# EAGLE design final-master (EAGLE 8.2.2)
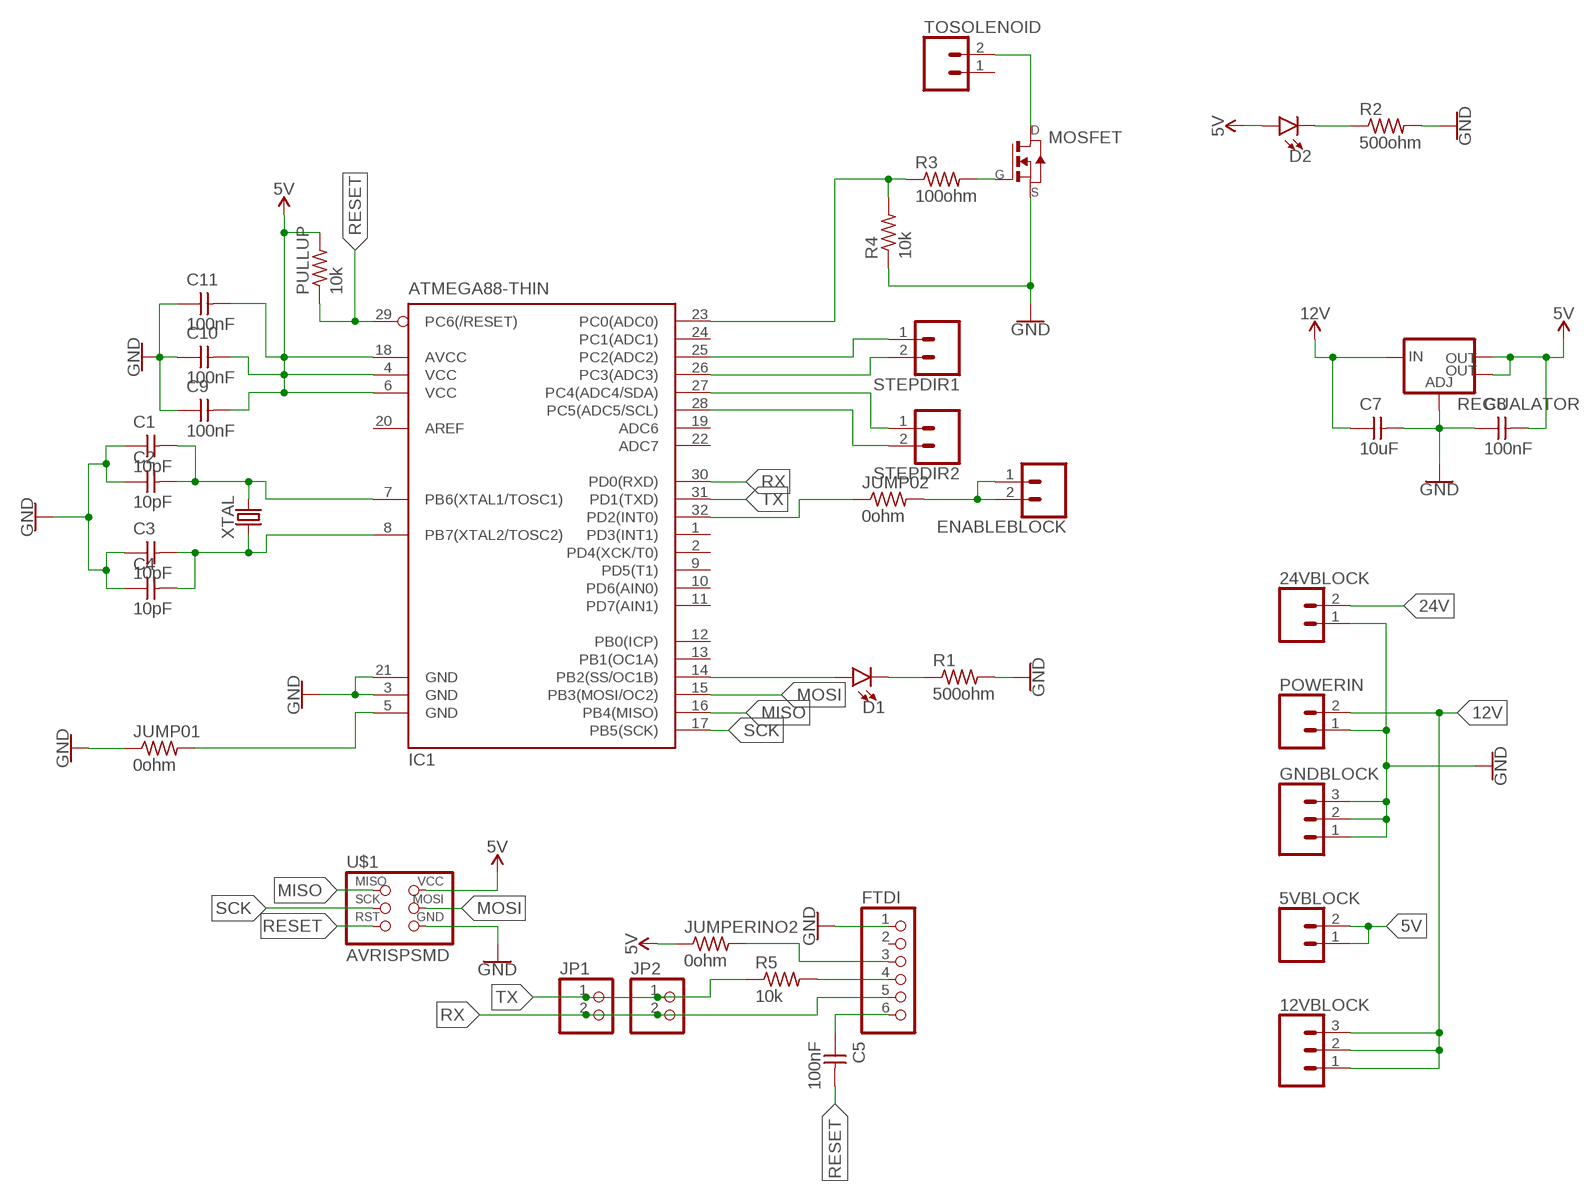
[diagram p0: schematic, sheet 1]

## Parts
5VBLOCK  CONN_023.5MM_LOCK  [SCREWTERMINAL-3.5MM-2_LOCK]
12VBLOCK  CONN_03SCREW_LOCK  [SCREWTERMINAL-3.5MM-3_LOCK.007S]
24VBLOCK  CONN_023.5MM_LOCK  [SCREWTERMINAL-3.5MM-2_LOCK]
C1  10pF  CAP-UNPOLARIZEDFAB  [C1206FAB]
C2  10pF  CAP-UNPOLARIZEDFAB  [C1206FAB]
C3  10pF  CAP-UNPOLARIZEDFAB  [C1206FAB]
C4  10pF  CAP-UNPOLARIZEDFAB  [C1206FAB]
C5  100nF  CAP-UNPOLARIZEDFAB  [C1206FAB]
C7  10uF  CAP-UNPOLARIZEDFAB  [C1206FAB]
C8  100nF  CAP-UNPOLARIZEDFAB  [C1206FAB]
C9  100nF  CAP-UNPOLARIZEDFAB  [C1206FAB]
C10  100nF  CAP-UNPOLARIZEDFAB  [C1206FAB]
C11  100nF  CAP-UNPOLARIZEDFAB  [C1206FAB]
D1  LED1206  [LED-1206]
D2  LED1206  [LED-1206]
ENABLEBLOCK  CONN_023.5MM_LOCK  [SCREWTERMINAL-3.5MM-2_LOCK]
FTDI  PINHD-1X6  [1X06]
GNDBLOCK  CONN_03SCREW_LOCK  [SCREWTERMINAL-3.5MM-3_LOCK.007S]
IC1  ATMEGA88-THIN  [TQFP32-08THIN]
JP1  PINHD-1X2  [1X02]
JP2  PINHD-1X2  [1X02]
JUMP01  0ohm  RES-US1206FAB  [R1206FAB]
JUMP02  0ohm  RES-US1206FAB  [R1206FAB]
JUMPERINO2  0ohm  RES-US1206FAB  [R1206FAB]
MOSFET  STN3NF06L  [SOT223]
POWERIN  CONN_023.5MM  [SCREWTERMINAL-3.5MM-2]
PULLUP  10k  RES-US1206FAB  [R1206FAB]
R1  500ohm  RES-US1206FAB  [R1206FAB]
R2  500ohm  RES-US1206FAB  [R1206FAB]
R3  100ohm  RES-US1206FAB  [R1206FAB]
R4  10k  RES-US1206FAB  [R1206FAB]
R5  10k  RES-US1206FAB  [R1206FAB]
REGUALATOR  V_REG_LM1117SOT223  [SOT223]
STEPDIR1  CONN_023.5MM_LOCK  [SCREWTERMINAL-3.5MM-2_LOCK]
STEPDIR2  CONN_023.5MM_LOCK  [SCREWTERMINAL-3.5MM-2_LOCK]
TOSOLENOID  CONN_023.5MM  [SCREWTERMINAL-3.5MM-2]
U$1  AVRISPSMD  [2X03SMD]
XTAL  CRYSTALSMD-HC49UP  [HC49UP]

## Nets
5V: 5VBLOCK.1 5VBLOCK.2 C8.2 C9.2 C10.2 C11.2 D2.A IC1.4(VCC) IC1.6(VCC) IC1.18(AVCC) JUMPERINO2.1 PULLUP.2 REGUALATOR.2(OUT) REGUALATOR.4(OUT) U$1.2(VCC)
12V: 12VBLOCK.1 12VBLOCK.2 12VBLOCK.3 C7.1 POWERIN.2 REGUALATOR.3(IN)
24V: 24VBLOCK.2
DIR1: IC1.26(PC3(ADC3)) STEPDIR1.2
DIR2: IC1.27(PC4(ADC4/SDA)) STEPDIR2.1
DRAIN: MOSFET.2(D) MOSFET.4(D) TOSOLENOID.2
ENABLEPIN: IC1.32(PD2(INT0)) JUMP02.1
GATE: MOSFET.1(G) R3.2
GND: 24VBLOCK.1 C1.1 C2.1 C3.1 C4.1 C7.2 C8.1 C9.1 C10.1 C11.1 FTDI.1 GNDBLOCK.1 GNDBLOCK.2 GNDBLOCK.3 IC1.3(GND) IC1.5(GND) IC1.21(GND) JUMP01.1 JUMP01.2 MOSFET.3(S) POWERIN.1 R1.2 R2.2 R4.1 REGUALATOR.1(ADJ) U$1.6(GND)
MISO: IC1.16(PB4(MISO)) U$1.1(MISO)
MOSI: IC1.15(PB3(MOSI/OC2)) U$1.4(MOSI)
N$1: C3.2 C4.2 IC1.8(PB7(XTAL2/TOSC2)) XTAL.1
N$2: C1.2 C2.2 IC1.7(PB6(XTAL1/TOSC1)) XTAL.2
N$3: IC1.23(PC0(ADC0)) R3.1 R4.2
N$4: ENABLEBLOCK.1 ENABLEBLOCK.2 JUMP02.2
N$6: D1.A IC1.14(PB2(SS/OC1B))
N$7: FTDI.3 JUMPERINO2.2
N$8: C5.1 FTDI.6
N$12: FTDI.4 R5.2
N$23: D2.C R2.1
N$26: D1.C R1.1
RESET: C5.2 IC1.29(PC6(/RESET)) PULLUP.1 U$1.5(RST)
RX: FTDI.5 IC1.30(PD0(RXD)) JP1.2 JP2.2
SCK: IC1.17(PB5(SCK)) U$1.3(SCK)
STEP1: IC1.25(PC2(ADC2)) STEPDIR1.1
STEP2: IC1.28(PC5(ADC5/SCL)) STEPDIR2.2
TX: IC1.31(PD1(TXD)) JP1.1 JP2.1 R5.1
Unconnected: FTDI.2 IC1.1(PD3(INT1)) IC1.2(PD4(XCK/T0)) IC1.9(PD5(T1)) IC1.10(PD6(AIN0)) IC1.11(PD7(AIN1)) IC1.12(PB0(ICP)) IC1.13(PB1(OC1A)) IC1.19(ADC6) IC1.20(AREF) IC1.22(ADC7) IC1.24(PC1(ADC1)) TOSOLENOID.1

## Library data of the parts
5VBLOCK 24VBLOCK ENABLEBLOCK POWERIN STEPDIR1 STEPDIR2 TOSOLENOID = SparkFun-Connectors:CONN_02: Multi connection point. Often used as Generic Header-pin footprint for 0.1 inch spaced/style header connections; PROD_ID: CONN-08399
12VBLOCK GNDBLOCK = SparkFun-Connectors:CONN_03: Multi connection point. Often used as Generic Header-pin footprint for 0.1 inch spaced/style header connections On any of the 0.1 inch spaced packages, you can populate with these: Break Away Headers - Straight (PRT-00116) Break Away Male Headers - Right Angle (PRT-00553) Female Headers (PRT-00115)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; PROD_ID: CONN-08288; SF_ID: PRT-08235
C1-C5 C7-C11 = 01fab:CAP-UNPOLARIZED
D1 D2 = SparkFun-LED:LED: LED (Generic)
FTDI = pinhead:PINHD-1X6: PIN HEADER
IC1 = 01fab:ATMEGA88-THIN
JP1 JP2 = pinhead:PINHD-1X2: PIN HEADER
JUMP01 JUMP02 JUMPERINO2 PULLUP R1-R5 = 01fab:RES-US: Resistor (US Symbol)
MOSFET = 01guercio:STN3NF06L
REGUALATOR = 01fab:V_REG_LM1117: Voltage Regulator LM1117 Standard adjustable voltage regulator but in SMD form. Spark Fun Electronics SKU : COM-00595; PROD_ID: VREG-08170
U$1 = 01fab:AVRISP
XTAL = SparkFun-Clocks:CRYSTAL: Crystals (Generic)

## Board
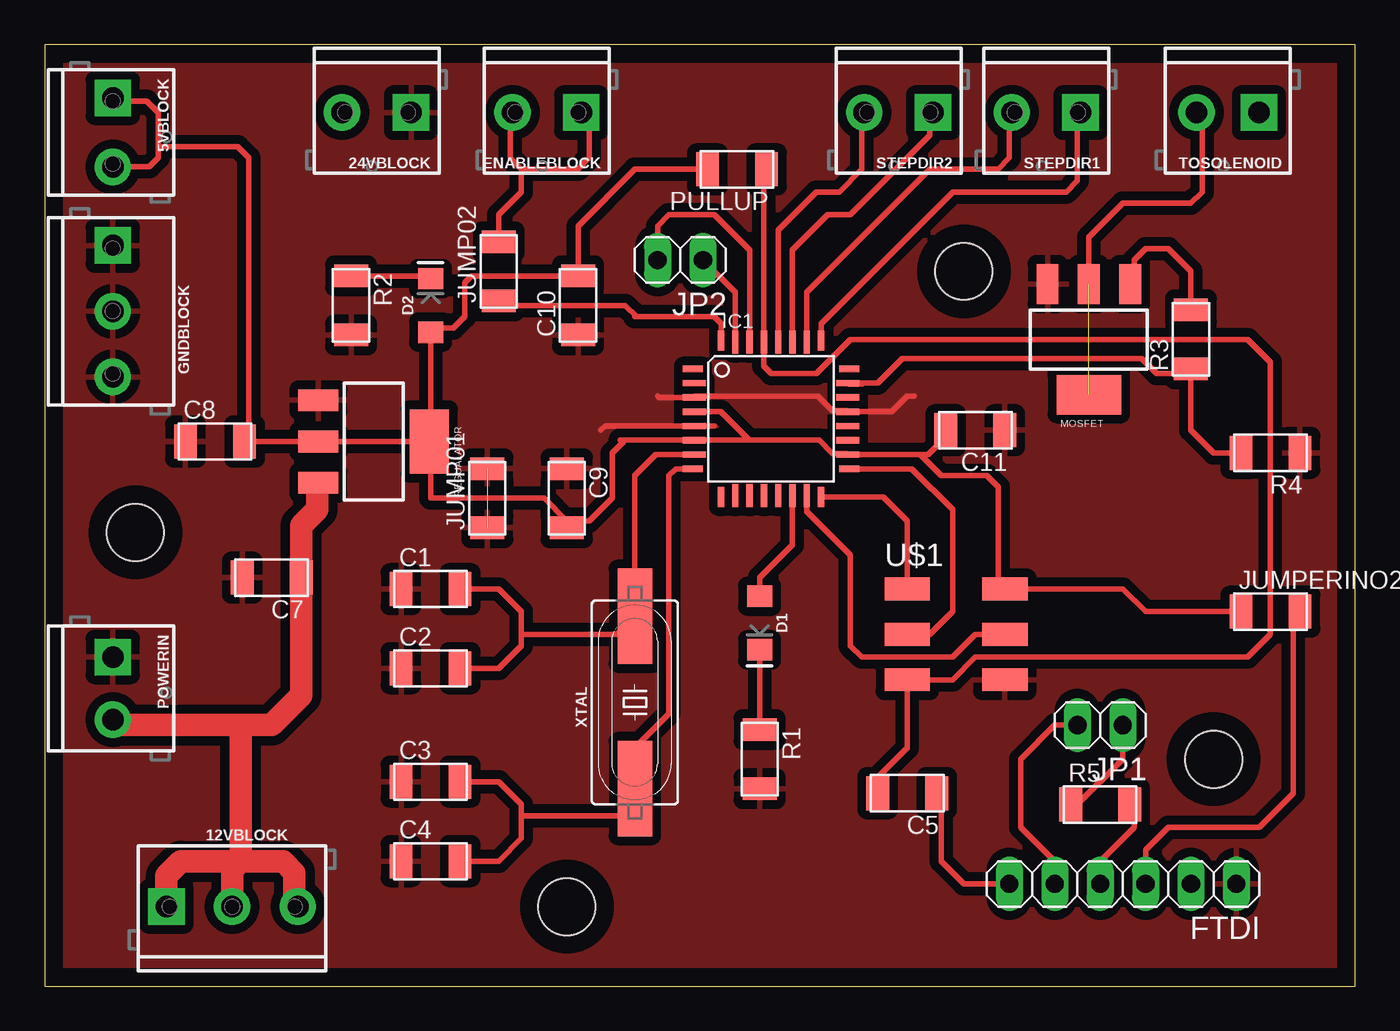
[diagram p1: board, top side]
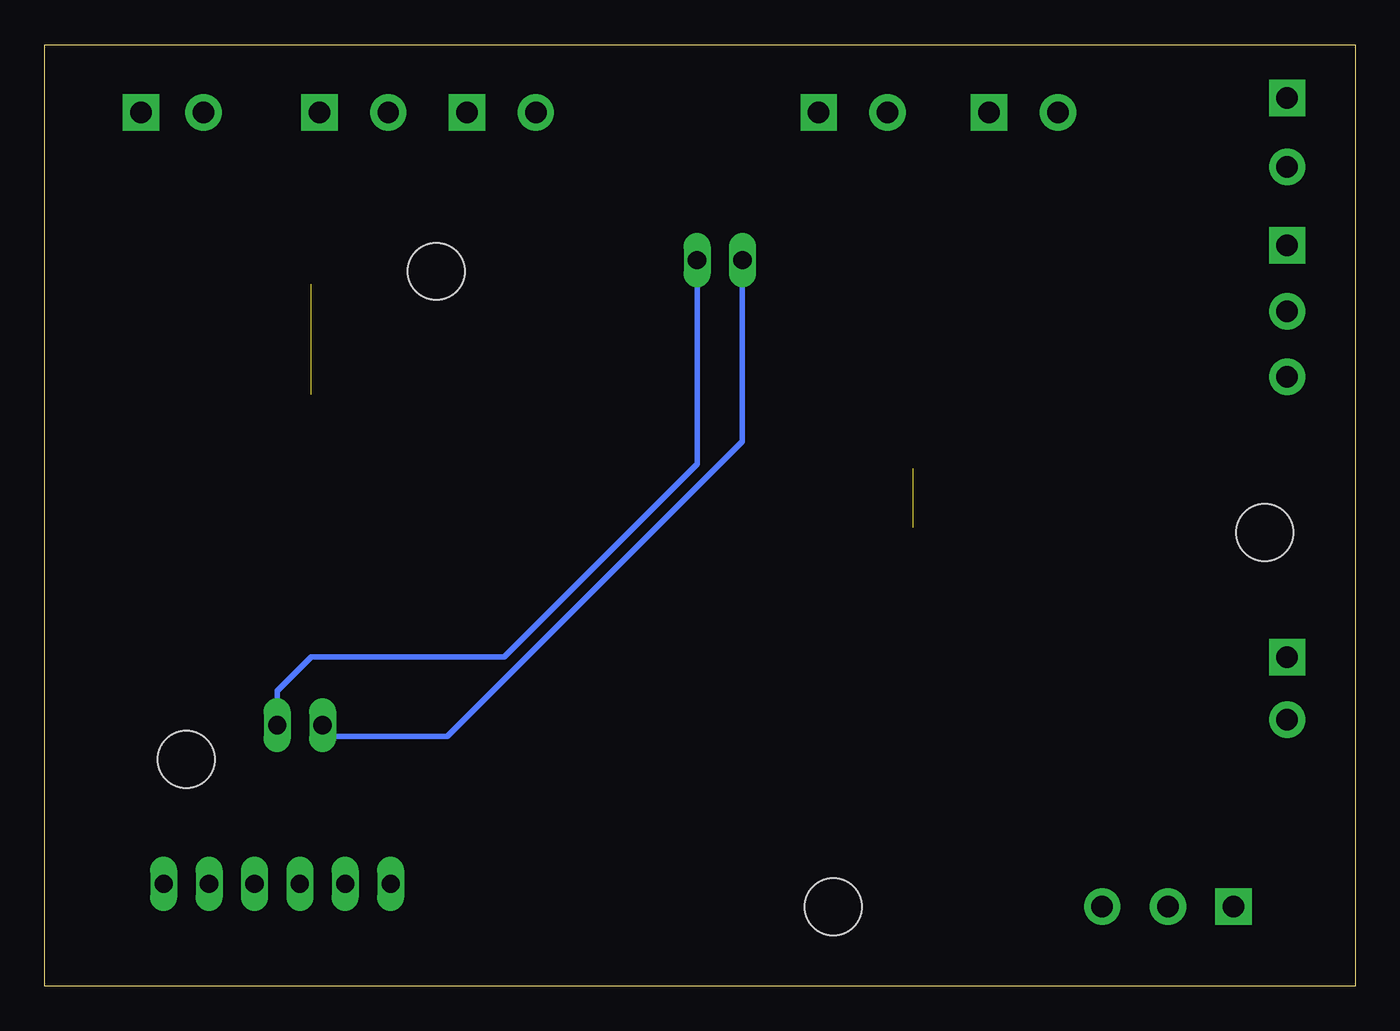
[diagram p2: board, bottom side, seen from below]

Size 73.33 x 52.7 mm. Coordinates in mm from the lower left corner, seen from the top.
Outline: 0,0 73.33,0 73.33,52.7 0,52.7 0,0
Copper layers (1*16): Top 0.035mm / dielectric 1.5mm / Bottom 0.035mm
Design rules "default *": minimum track width 12mil, minimum drill 0.35mm, track to track 16mil, track to pad 16mil, pad to pad 16mil, via to via 16mil, smd to smd 16mil, copper to edge 40mil, drill to drill 6mil, minimum pad ring 10mil, minimum via ring 8mil, stop-mask expansion 4mil, vias tented up to drill 0mil, thermal gap 20mil
Holes 3.2 mm at 51.44,40.01 29.21,4.45 65.41,12.7 5.08,25.4

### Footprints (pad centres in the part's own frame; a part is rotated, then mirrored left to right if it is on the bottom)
SCREWTERMINAL-3.5MM-2_LOCK = drill 1.2 pad 2.032 square: 1 -0.178,0 | drill 1.2 pad 2.032: 2 3.678,0
SCREWTERMINAL-3.5MM-3_LOCK.007S = drill 1.2 pad 2.032 square: 1 -0.178,0 | drill 1.2 pad 2.032: 2 3.5,0; 3 7.178,0
C1206FAB = smd 1.27 x 1.905: 1 -1.651,0; 2 1.651,0
LED-1206 = smd 1.2 x 1.4: A -1.5,0; C 1.5,0
1X06 = drill 1.016 long: 1 -6.35,0; 2 -3.81,0; 3 -1.27,0; 4 1.27,0; 5 3.81,0; 6 6.35,0
TQFP32-08THIN = smd 1.118 x 0.356: 1 -4.369,2.8; 8 -4.369,-2.8; 17 4.369,-2.8; 24 4.369,2.8 | smd 1.27 x 0.356: 2 -4.293,2; 3 -4.293,1.2; 4 -4.293,0.4; 5 -4.293,-0.4; 6 -4.293,-1.2; 7 -4.293,-2; 18 4.293,-2; 19 4.293,-1.2; 20 4.293,-0.4; 21 4.293,0.4; 22 4.293,1.2; 23 4.293,2 | smd 0.356 x 1.118: 9 -2.8,-4.369; 16 2.8,-4.369; 25 2.8,4.369; 32 -2.8,4.369 | smd 0.356 x 1.27: 10 -2,-4.293; 14 1.2,-4.293; 15 2,-4.293; 26 2,4.293; 27 1.2,4.293; 31 -2,4.293 | smd 0.35 x 1.27: 11 -1.2,-4.293; 12 -0.4,-4.293; 13 0.4,-4.293; 28 0.4,4.293; 29 -0.4,4.293; 30 -1.2,4.293
1X02 = drill 1.016 long: 1 -1.27,0; 2 1.27,0
R1206FAB = smd 1.27 x 1.905: 1 -1.651,0; 2 1.651,0
SOT223 = smd 1.219 x 2.235: 1 -2.311,-3.099; 2 0,-3.099; 3 2.311,-3.099 | smd 3.6 x 2.2: 4 0,3.099
SCREWTERMINAL-3.5MM-2 = drill 1.2 pad 2.032 square: 1 0,0 | drill 1.2 pad 2.032: 2 3.5,0
2X03SMD = smd 2.54 x 1.27: 1 -2.54,2.54; 2 2.92,2.54; 3 -2.54,0; 4 2.92,0; 5 -2.54,-2.54; 6 2.92,-2.54
HC49UP = smd 5.334 x 1.93: 1 -4.826,0; 2 4.826,0

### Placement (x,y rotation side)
5VBLOCK  3.81,49.53 270 top
12VBLOCK  6.99,4.45 0 top
24VBLOCK  20.32,48.9 180 top
C1  21.59,22.23 0 top
C2  21.59,17.78 0 top
C3  21.59,11.43 0 top
C4  21.59,6.99 0 top
C5  48.26,10.79 180 top
C7  12.7,22.86 180 top
C8  9.53,30.48 0 top
C9  29.21,27.3 270 top
C10  29.84,38.1 90 top
C11  52.07,31.11 180 top
D1  40.01,20.32 270 top
D2  21.59,38.1 90 top
ENABLEBLOCK  29.84,48.9 180 top
FTDI  60.33,5.71 180 top
GNDBLOCK  3.81,41.27 270 top
IC1  40.64,31.75 0 top
JP1  59.05,14.61 180 top
JP2  35.56,40.64 180 top
JUMP01  24.77,27.3 90 top
JUMP02  25.4,40.01 90 top
JUMPERINO2  68.58,20.95 0 top
MOSFET  58.42,36.2 180 top
POWERIN  3.81,18.41 270 top
PULLUP  38.73,45.72 180 top
R1  40.01,12.7 270 top
R2  17.14,38.1 270 top
R3  64.14,36.2 90 top
R4  68.58,29.84 180 top
R5  59.05,10.16 0 top
REGUALATOR  18.41,30.48 270 top
STEPDIR1  57.78,48.9 180 top
STEPDIR2  49.53,48.9 180 top
TOSOLENOID  67.94,48.9 180 top
U$1  50.8,19.68 0 top
XTAL  33.02,15.88 90 top

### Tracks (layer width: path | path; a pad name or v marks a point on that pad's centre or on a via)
5V
  Top 0.305: 32.2,30.55 32.38,30.55 | 32.38,30.55 IC1.6 39.41,30.55 | REGUALATOR.4 21.59,30.4 21.59,27.3 27.94,27.3 29.21,26.04 C9.2 29.59,26.04 30.48,26.04 31.75,27.3 31.75,29.84 32.38,30.48 32.38,30.55 | 39.41,30.55 43.33,30.55 44.07,29.81 44.87,29.81 IC1.18 48.99,29.75 | 48.99,29.75 49.44,29.75 50.16,30.48 50.16,30.86 C11.2 | REGUALATOR.4 21.59,30.56 D2.A 21.82,36.83 22.86,36.83 23.5,37.47 23.5,39.37 23.88,39.75 C10.2 29.84,42.55 33.02,45.72 PULLUP.2 | 48.99,29.75 50.16,28.57 52.7,28.57 53.34,27.94 53.34,22.61 U$1.2 60.33,22.23 61.59,20.95 JUMPERINO2.1 | 5VBLOCK.2 5.85,45.85 6.35,46.35 6.35,46.99 | 6.35,46.99 6.35,48.9 5.71,49.53 3.99,49.53 5VBLOCK.1 | 6.35,46.99 10.79,46.99 11.43,46.35 11.43,30.73 C8.2 REGUALATOR.2 REGUALATOR.4 | IC1.4 37.81,32.15 39.41,30.55
12V
  Top 1.27: 10.85,14.61 12.7,14.61 14.35,16.26 C7.1 14.35,25.78 15.24,26.67 15.24,28.09 REGUALATOR.3 | 10.85,14.61 4.12,14.61 POWERIN.2 | 12VBLOCK.1 6.81,6.17 7.62,6.99 10.98,6.99 | 12VBLOCK.3 13.97,4.64 13.97,6.35 13.34,6.99 10.98,6.99 | 12VBLOCK.2 10.48,6.49 10.98,6.99 | 10.98,6.99 10.98,14.47 10.85,14.61
DIR1
  Top 0.305: IC1.26 42.64,38.83 49.53,45.72 53.34,45.72 53.98,46.35 53.98,48.76 STEPDIR1.2
DIR2
  Top 0.305: IC1.27 41.84,41.2 43.81,43.18 45.09,43.18 49.53,47.62 49.53,48.72 STEPDIR2.1
DRAIN  (1 unrouted)
  Top 0.305: MOSFET.2 58.42,41.91 60.33,43.81 64.14,43.81 64.77,44.45 64.77,48.57 TOSOLENOID.2
ENABLEPIN
  Top 0.305: IC1.32 37.84,37.09 37.47,37.47 33.12,37.47 | 33.12,37.47 33.02,37.47 | JUMP02.1 25.65,38.1 32.48,38.1 33.12,37.47
GATE
  Top 0.305: R3.2 64.14,40.01 62.87,41.27 61.59,41.27 60.96,40.64 60.96,39.52 MOSFET.1
GND  (1 unrouted)
  Top 0.305: 48.64,33.02 48.26,33.02 47.39,32.15 IC1.21 44.87,32.21 44.07,32.21 43.26,33.02 37.22,33.02 37.21,33.01 36.41,33.01 IC1.3 34.36,32.95 34.29,33.02 | 37.45,31.35 IC1.5 31.35,31.35 31.11,31.11
  pour Top (isolate 0.508): -2.54,-2.54 102.23,-2.54 102.87,-1.91 102.87,82.55 103.5,83.19 -2.54,83.19
MISO
  Top 0.305: IC1.16 46.91,27.38 48.26,26.04 U$1.1
MOSI
  Top 0.305: IC1.15 42.64,26.57 45.09,24.13 45.09,19.05 45.72,18.41 50.8,18.41 52.07,19.68 U$1.4
N$1
  Top 0.305: IC1.8 35.3,28.95 34.92,28.57 34.92,15.24 33.02,13.34 XTAL.1 33.02,9.53 26.67,9.53 | C4.2 25.4,6.99 26.67,8.26 26.67,9.53 | 26.67,9.53 26.67,10.16 25.4,11.43 C3.2
N$2
  Top 0.305: IC1.7 34.2,29.75 33.02,28.57 XTAL.2 32,19.68 26.67,19.68 | C1.2 25.4,22.23 26.67,20.95 26.67,19.68 | 26.67,19.68 26.67,19.05 25.4,17.78 C2.2
N$3
  Top 0.305: 45.75,33.69 45,33.69 IC1.23 46.6,33.75 47.99,35.14 61.38,35.14 62.23,34.29 63.88,34.29 R3.1 64.14,31.11 65.41,29.84 R4.2
N$4
  Top 0.305: 26.84,45.72 26.67,45.72 26.04,46.35 26.04,48.76 ENABLEBLOCK.2 | 26.84,45.72 29.84,45.72 30.48,46.35 30.48,48.44 ENABLEBLOCK.1 | 26.84,45.72 26.67,45.55 26.67,44.45 25.4,43.18 JUMP02.2
N$6
  Top 0.305: IC1.14 41.84,24.7 40.01,22.86 D1.A
N$7
  Top 0.305: FTDI.3 61.59,7.62 62.87,8.89 67.94,8.89 69.85,10.79 69.85,20.57 JUMPERINO2.2
N$8
  Top 0.305: FTDI.6 51.44,5.71 50.16,6.99 50.16,10.54 C5.1
N$12
  Top 0.305: FTDI.4 59.05,6.99 60.96,8.89 60.96,9.91 R5.2
N$23
  Top 0.305: R2.1 21.44,39.75 D2.C
N$26
  Top 0.305: D1.C R1.1
RESET
  Top 0.305: PULLUP.1 40.24,45.57 IC1.29 40.24,34.69 40.64,34.29 43.18,34.29 45.09,36.2 67.31,36.2 68.58,34.92 68.58,19.68 67.31,18.41 52.07,18.41 50.8,17.14 U$1.5 48.26,13.34 46.61,11.68 C5.2
RX
  Top 0.305: FTDI.5 56.52,6.99 54.61,8.89 54.61,12.7 56.52,14.61 JP1.2 | IC1.30 39.44,41.2 37.47,43.18 34.92,43.18 34.29,42.55 JP2.2
  Bottom 0.305: JP2.2 34.29,30.48 50.8,13.97 57.15,13.97 JP1.2
SCK
  Top 0.305: IC1.17 48.52,28.95 50.8,26.67 50.8,20.95 49.53,19.68 U$1.3
STEP1
  Top 0.305: IC1.25 43.44,37.09 50.8,44.45 57.15,44.45 57.78,45.09 57.78,48.72 STEPDIR1.1
STEP2
  Top 0.305: IC1.28 41.04,42.31 43.18,44.45 44.45,44.45 45.72,45.72 45.72,48.76 STEPDIR2.2
TX
  Top 0.305: 38.64,37.3 IC1.31 38.64,38.83 JP2.1 | R5.1 57.78,10.16 60.33,12.7 JP1.1
  Bottom 0.305: JP1.1 60.33,16.51 58.42,18.41 47.62,18.41 36.83,29.21 JP2.1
